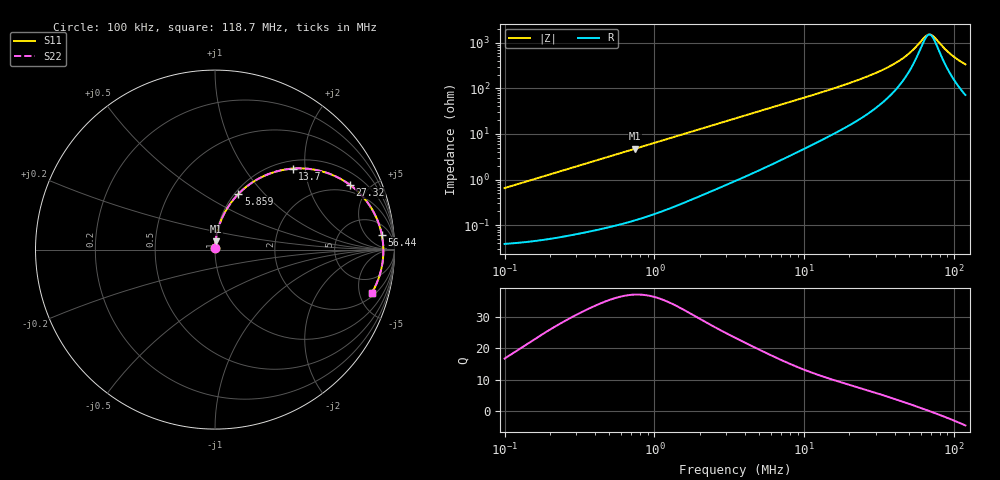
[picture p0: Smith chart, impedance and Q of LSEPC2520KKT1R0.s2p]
! LSEPC2520KKT1R0  S-PARAMETER MODEL  ( General Type )
! Model Generated by TAIYO YUDEN Corporation (http://www.ty-top.com)
! Version 1.0
! TAIYO YUDEN Control No. 190603NI43SB-FBB
! Copyright(c) 2019 TAIYO YUDEN CO.,LTD. All Rights Reserved.
! Product Description (link to TY-COMPAS)
! https://ds.yuden.co.jp/TYCOMPAS/or/detail?pn=LSEPC2520KKT1R0M&u=M
! Products Name : Inductors
! Characteristics :
!  Inductance : 1.0 uH , SRF(min) : -Hz , DC Resistance(max) : 0.039 Ohm
!  Rated Current : Saturation :4400 mA , Temp Rise : 3800 mA (40 degC)
!  Case Size : 2.5 x 2.0 / 0.098 x 0.079 [mm/inch] , Thickness : 1 / 0.039 [mm/inch]
!  (Conditions: Temperature = 25 degC , DC Bias Current/Voltage = 0A / 0V)
! External Node Assignments :
!  1  o---GGG---o  2
! GND o---------o GND
! Frequency Range : 0.1MHz  -  118.695536MHz  [ 402 STEP ]
# MHz S RI R 50
! Freq[MHz].  S11 Real  S11 Imag  S21 Real  S21 Imag  S12 Real  S12 Imag  S22 Real  S22 Imag
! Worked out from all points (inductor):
!   401 points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, 100 kHz to 118.7 MHz, reference 50 ohm
!   read as one part in series: L = 1.03 uH near 103.6 kHz
!   highest Q = 37.1 at 738.8 kHz (marker M1), where L = 1.01 uH
!   self-resonance near 68.21 MHz
!   S11 on the Smith chart (normalised r, x): 100 kHz: 1.00, +0.01; 5.859 MHz: 1.04, +0.73; 13.7 MHz: 1.16, +1.71; 27.32 MHz: 1.59, +3.77; 56.44 MHz: 11, +14; 118.7 MHz: 2.42, -6.54
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0.1  0.000429 0.00648  0.9996 -0.00648  0.9996 -0.00648  0.000429 0.00648
0.327316  0.00111 0.021  0.9989 -0.021  0.9989 -0.021  0.00111 0.021
0.738801  0.00347 0.0469  0.9965 -0.0469  0.9965 -0.0469  0.00347 0.0469
1.07136  0.00647 0.0675  0.9935 -0.0675  0.9935 -0.0675  0.00647 0.0675
1.990437  0.0196 0.1226  0.9804 -0.1226  0.9804 -0.1226  0.0196 0.1226
3.445222  0.0524 0.2024  0.9476 -0.2024  0.9476 -0.2024  0.0524 0.2024
5.85868  0.1307 0.3104  0.8693 -0.3104  0.8693 -0.3104  0.1307 0.3104
8.056554  0.2159 0.3794  0.7841 -0.3794  0.7841 -0.3794  0.2159 0.3794
11.27678  0.3434 0.4356  0.6566 -0.4356  0.6566 -0.4356  0.3434 0.4356
13.70036  0.4319 0.4512  0.5681 -0.4512  0.5681 -0.4512  0.4319 0.4512
19.17642  0.595 0.4363  0.405 -0.4363  0.405 -0.4363  0.595 0.4363
27.32054  0.7524 0.3603  0.2476 -0.3603  0.2476 -0.3603  0.7524 0.3603
36.91074  0.8532 0.258  0.1468 -0.258  0.1468 -0.258  0.8532 0.258
46.45921  0.9042 0.1658  0.0958 -0.1658  0.0958 -0.1658  0.9042 0.1658
56.44413  0.9292 0.0828  0.0708 -0.0828  0.0708 -0.0828  0.9292 0.0828
65.02906  0.9372 0.021  0.0628 -0.021  0.0628 -0.021  0.9372 0.021
69.79942  0.9381 -0.0102  0.0619 0.0102  0.0619 0.0102  0.9381 -0.0102
73.60547  0.9373 -0.0336  0.0627 0.0336  0.0627 0.0336  0.9373 -0.0336
84.80057  0.9293 -0.0959  0.0707 0.0959  0.0707 0.0959  0.9293 -0.0959
94.30078  0.9175 -0.1424  0.0825 0.1424  0.0825 0.1424  0.9175 -0.1424
106.7377  0.8973 -0.1957  0.1027 0.1957  0.1027 0.1957  0.8973 -0.1957
118.6955  0.8742 -0.2402  0.1258 0.2402  0.1258 0.2402  0.8742 -0.2402
